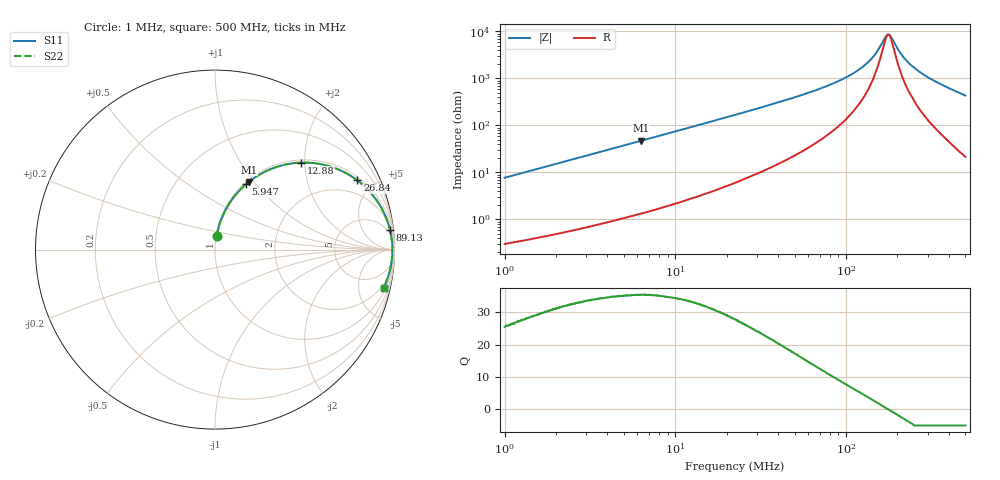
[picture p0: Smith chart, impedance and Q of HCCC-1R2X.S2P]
!s-Parameter Generated by FASTRON Sdn. Bhd.
!FASTRON P/N : HCCC-1R2X
!Keysight Technologies,E4991B,MY54100416,A.01.15
!Date: Mon Apr 06 15:43:46 2026
!Version  : Rev00 Mon Apr 06 15:43:46 2026
!Data & Calibration Information:
!PortZ  Port1:50+j0  Port2:50+j0
!When reading, reference impedance value at option line is always used.
!Remarks : This data is being provided solely for informational purposes.
!Freq	S11	S21	S12	S22
# Hz S dB R 50
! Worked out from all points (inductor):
!   1601 points, 1 MHz to 500 MHz, reference 50 ohm
!   read as one part in series: L = 1.22 uH near 1.032 MHz
!   highest Q = 35.4 at 6.303 MHz (marker M1), where L = 1.19 uH
!   self-resonance near 176.9 MHz
!   S11 on the Smith chart (normalised r, x): 1 MHz: 1.01, +0.15; 5.947 MHz: 1.03, +0.89; 12.88 MHz: 1.06, +1.92; 26.84 MHz: 1.16, +4.03; 89.13 MHz: 3, +17; 500 MHz: 1.43, -8.61
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1000000  -22.32 83.4  -0.05 -4.4  -0.05 -4.4  -22.32 83.4
2820919  -13.67 76.3  -0.25 -12.0  -0.25 -12.0  -13.67 76.3
5946577  -7.91 64.7  -0.87 -23.7  -0.87 -23.7  -7.91 64.7
6303327  -7.50 63.4  -0.97 -24.9  -0.97 -24.9  -7.50 63.4
7957584  -5.95 58.1  -1.42 -30.3  -1.42 -30.3  -5.95 58.1
1.288105e7  -3.33 45.3  -2.96 -43.0  -2.96 -43.0  -3.33 45.3
2.236068e7  -1.47 30.4  -5.92 -57.6  -5.92 -57.6  -1.47 30.4
2.683906e7  -1.09 25.9  -7.17 -61.8  -7.17 -61.8  -1.09 25.9
3.988656e7  -0.56 17.8  -10.29 -69.4  -10.29 -69.4  -0.56 17.8
6.307767e7  -0.27 10.6  -14.65 -75.3  -14.65 -75.3  -0.27 10.6
8.912629e7  -0.16 6.5  -18.83 -77.3  -18.83 -77.3  -0.16 6.5
1.112133e8  -0.13 4.3  -22.45 -76.6  -22.45 -76.6  -0.13 4.3
1.319406e8  -0.11 2.7  -26.41 -73.2  -26.41 -73.2  -0.11 2.7
1.494024e8  -0.10 1.5  -30.74 -64.9  -30.74 -64.9  -0.10 1.5
1.711582e8  -0.10 0.3  -37.99 -23.8  -37.99 -23.8  -0.10 0.3
1.77937e8  -0.10 -0.1  -38.77 4.6  -38.77 4.6  -0.10 -0.1
1.842672e8  -0.10 -0.4  -37.62 29.1  -37.62 29.1  -0.10 -0.4
2.022705e8  -0.10 -1.2  -32.27 60.8  -32.27 60.8  -0.10 -1.2
2.160773e8  -0.10 -1.9  -29.27 68.6  -29.27 68.6  -0.10 -1.9
2.573461e8  -0.12 -3.6  -23.96 76.0  -23.96 76.0  -0.12 -3.6
3.364424e8  -0.16 -6.6  -18.71 77.7  -18.71 77.7  -0.16 -6.6
5e8  -0.32 -12.9  -13.01 74.3  -13.01 74.3  -0.32 -12.9
